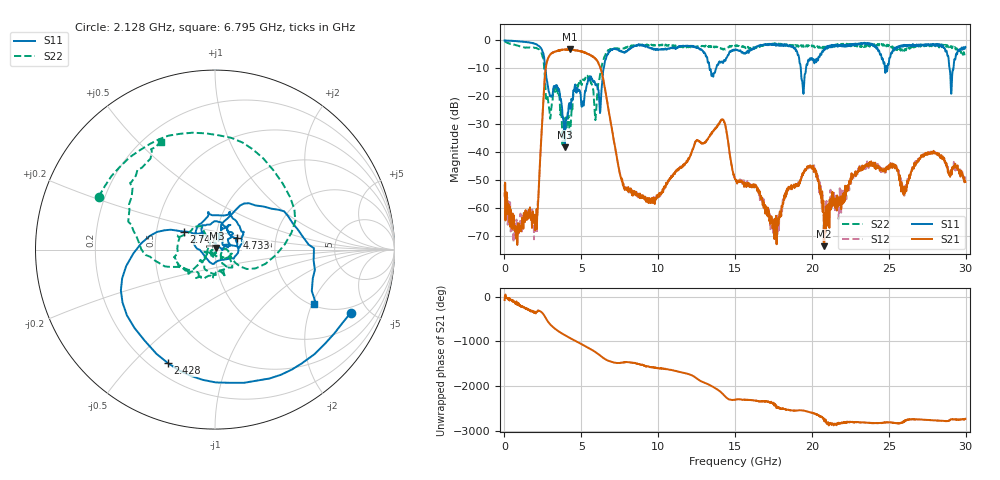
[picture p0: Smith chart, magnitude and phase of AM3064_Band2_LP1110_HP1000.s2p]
# Hz S DB R 50.0
!freq dBS11 angS11 dBS21 angS21 dBS12 angS12 dBS22 angS22
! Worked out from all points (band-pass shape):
!   1600 points, 10 MHz to 29.98 GHz, reference 50 ohm
!   highest |S21| = -3.20 dB at 4.246 GHz (marker M1); lowest = -73.6 dB at 20.8 GHz (marker M2)
!   |S21| within 3 dB of the highest: 2.854 GHz to 5.845 GHz (2.992 GHz wide, 68.8 % of centre)
!   lowest |S11| = -38.2 dB at 3.927 GHz (marker M3), VSWR 1.03, Z = 50.8 + j0.945 ohm
!   |S11| at or under -10 dB: 2.664 GHz to 6.453 GHz (3.79 GHz wide, 83.1 % of centre); 13.34 GHz to 13.76 GHz (422.7 MHz wide, 3.12 % of centre); 19.27 GHz to 19.61 GHz (341.6 MHz wide, 1.76 % of centre)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
!   |S22| runs from -37.3 to -0.3 dB; largest |S21 - S12| = 0.018
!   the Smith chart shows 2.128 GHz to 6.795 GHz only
!   S11 on the Smith chart (normalised r, x): 2.128 GHz: 1.65, -3.82; 2.428 GHz: 0.27, -0.64; 2.747 GHz: 0.69, +0.14; 4.733 GHz: 1.27, +0.17; 6.795 GHz: 2.08, -2.08
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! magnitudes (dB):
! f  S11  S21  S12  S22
! 10 MHz  0.0  -54.7  -51.5  -0.3
! 703.5 MHz  -0.2  -68.3  -68.1  -1.6
! 2.128 GHz  -1.6  -62.9  -60.3  -2.9
! 2.428 GHz  -3.3  -31.2  -31.0  -4.8
! 2.747 GHz  -14.0  -8.1  -8.0  -20.4
! 3.927 GHz  -38.2  -3.4  -3.3  -31.1
! 4.246 GHz  -22.7  -3.2  -3.2  -35.0
! 4.733 GHz  -17.0  -3.7  -3.6  -16.1
! 5.015 GHz  -23.5  -4.0  -3.9  -15.9
! 5.933 GHz  -16.1  -6.6  -6.7  -27.7
! 6.795 GHz  -4.0  -25.6  -25.6  -3.4
! 7.807 GHz  -4.2  -52.5  -52.6  -2.9
! 10 GHz  -3.4  -55.8  -55.6  -1.8
! 14.14 GHz  -7.7  -28.4  -28.5  -3.0
! 15 GHz  -3.2  -49.6  -49.7  -1.9
! 17.61 GHz  -1.7  -67.8  -67.3  -1.1
! 19.99 GHz  -6.3  -45.2  -45.4  -1.8
! 20.8 GHz  -3.0  -73.6  -59.6  -2.5
! 25 GHz  -8.4  -44.7  -45.1  -1.6
! 28.28 GHz  -1.4  -41.1  -41.1  -2.6
! 29.08 GHz  -17.7  -48.0  -46.8  -2.5
! 29.98 GHz  -2.4  -50.6  -50.5  -4.6
